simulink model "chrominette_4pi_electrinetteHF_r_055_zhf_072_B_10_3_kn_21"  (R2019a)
settings: Solver=VariableStepAuto  StartTime=0.0  StopTime=2329176.80  FixedStep=0.2  RelTol=1e-6

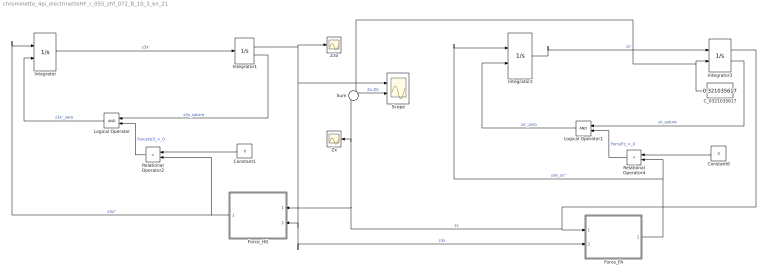
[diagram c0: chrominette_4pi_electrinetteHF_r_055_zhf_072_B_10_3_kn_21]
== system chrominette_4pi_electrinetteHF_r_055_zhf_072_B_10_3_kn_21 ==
  C_0321035617 : Constant  Value=0.321035617
  Constant1 : Constant  Value=0
  Constant6 : Constant  Value=0
  Force_FA : Subsystem
  Force_HG : Subsystem
  Integrator : Integrator  ExternalReset=level
  Integrator1 : Integrator  LimitOutput=on  UpperSaturationLimit=0  ShowSaturationPort=on  ZeroCross=off
  Integrator2 : Integrator  ExternalReset=level
  Integrator3 : Integrator  InitialConditionSource=external  LimitOutput=on  LowerSaturationLimit=0.321035617  ShowSaturationPort=on  ZeroCross=off
  Logical Operator : Logic  AllPortsSameDT=off  OutDataTypeStr=boolean
  Logical Operator1 : Logic  AllPortsSameDT=off  OutDataTypeStr=boolean
  Relational Operator2 : RelationalOperator  Operator=<  OutDataTypeStr=boolean  RndMeth=Simplest
  Relational Operator4 : RelationalOperator  Operator=>  OutDataTypeStr=boolean  RndMeth=Simplest
  Scope : Scope  NumInputPorts=2
  Sum : Sum  Inputs=-+
  Z3x : Scope
  Zx : Scope
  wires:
  Integrator/1 -> Integrator1/1  "z3x'"
  Integrator1/1 -> Scope/1, Force_FA/2(In2), Force_HG/2(In2), Z3x/1  "z3x"
  Force_HG/1(Out1) -> Relational Operator2/2, Integrator/1  "z3x''"
  Constant1/1 -> Relational Operator2/1
  Relational Operator2/1 -> Logical Operator/2  "ForceHz3_>_0"
  Constant6/1 -> Relational Operator4/1
  Integrator3/1 -> Force_HG/1(In1), Zx/1, Sum/2, Force_FA/1(In1)  "zx"
  Logical Operator1/1 -> Integrator2/2  "zx'_zero"
  Relational Operator4/1 -> Logical Operator1/2  "ForceFz_<_0"
  C_0321035617/1 -> Integrator3/2, Sum/1
  Force_FA/1(Out1) -> Integrator2/1, Relational Operator4/2  "pre_zx''"
  Integrator1/2 -> Logical Operator/1  "z3x_sature"
  Logical Operator/1 -> Integrator/2  "z3x'_zero"
  Integrator3/2 -> Logical Operator1/1  "zx_sature"
  Integrator2/1 -> Integrator3/1  "zx'"
  Sum/1 -> Scope/2  "Zx-Z0"

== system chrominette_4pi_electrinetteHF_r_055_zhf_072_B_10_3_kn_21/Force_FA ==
  In1 : Inport
  In2 : Inport  Port=2
  Add26 : Sum  Inputs=-+
  F_AG : Subsystem
  F_AH : Subsystem
  F_AI : Subsystem
  F_AJ : Subsystem
  F_FG : Subsystem
  F_FH : Subsystem
  F_FI : Subsystem
  F_FJ : Subsystem
  Scope14 : Scope
  Sum1 : Sum  Inputs=|+|-|+|-|-|+|-|+
  Z0_1 : Constant  Value=0.321035617
  Out1 : Outport
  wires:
  Sum1/1 -> Scope14/1, Out1/1  "pre_zx''"
  In1/1 -> F_AI/1(In1), F_AJ/1(In1), F_AG/1(In1), F_AH/1(In1), F_FH/1(In1), F_FG/1(In1), F_FJ/1(In1), F_FI/1(In1)
  F_FG/1(Out1) -> Sum1/5
  F_FI/1(Out1) -> Sum1/1
  Z0_1/1 -> Add26/2  "Z0"
  In2/1 -> Add26/1  "z3"
  Add26/1 -> F_FH/2(In2), F_AG/2(In2), F_FG/2(In2), F_AH/2(In2)  "z0 - z3"
  F_AI/1(Out1) -> Sum1/2
  F_FJ/1(Out1) -> Sum1/3
  F_AJ/1(Out1) -> Sum1/4
  F_AH/1(Out1) -> Sum1/8
  F_FH/1(Out1) -> Sum1/7
  F_AG/1(Out1) -> Sum1/6

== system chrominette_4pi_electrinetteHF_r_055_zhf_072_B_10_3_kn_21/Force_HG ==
  In1 : Inport
  In2 : Inport  Port=2
  F_HA : Subsystem
  F_HF : Subsystem
  F_HI : Subsystem
  F_HJ : Subsystem
  Scope : Scope
  Sum : Sum  Inputs=|+|-|+|-
  Out1 : Outport
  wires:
  In2/1 -> F_HJ/2(In2), F_HI/2(In2), F_HF/2(In2), F_HA/2(In2)
  In1/1 -> F_HJ/1(In1), F_HI/1(In1), F_HF/1(In1), F_HA/1(In1)
  Sum/1 -> Out1/1, Scope/1  "pre_z3x''"
  F_HA/1(Out1) -> Sum/1
  F_HF/1(Out1) -> Sum/2
  F_HI/1(Out1) -> Sum/3
  F_HJ/1(Out1) -> Sum/4

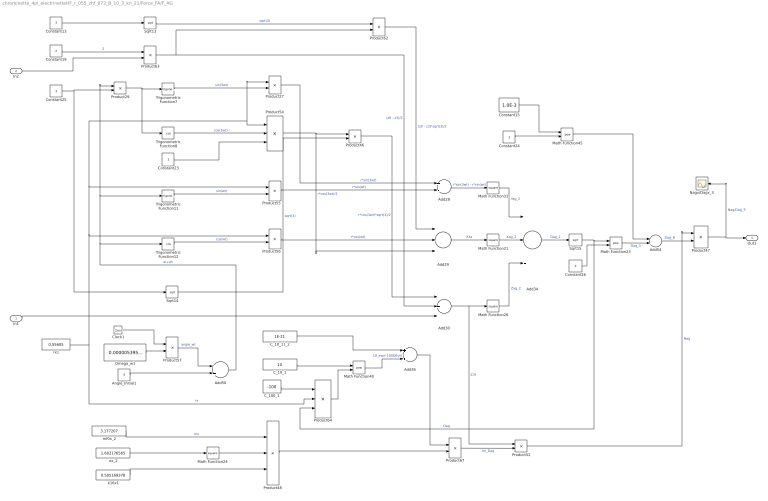
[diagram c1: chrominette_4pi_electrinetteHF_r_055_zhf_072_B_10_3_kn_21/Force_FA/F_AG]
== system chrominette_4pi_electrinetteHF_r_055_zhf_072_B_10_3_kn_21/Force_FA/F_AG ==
  In1 : Inport
  In2 : Inport  Port=2
  Add28 : Sum  Inputs=+-
  Add29 : Sum  Inputs=-++
  Add30 : Sum  Inputs=+++
  Add34 : Sum  Inputs=+++
  Add36 : Sum
  Add50 : Sum
  Add54 : Sum
  Angle_Initial1 : Constant  Value=0
  C_100_1 : Constant  Value=-100
  C_10_1 : Constant  Value=10
  C_10_11_2 : Constant  Value=1E-21
  Clock1 : Clock
  Constant{13,24..26} (4 alike) : Constant  Value=3
  Constant15 : Constant  Value=1.0E-3
  Constant19 : Constant  Value=2
  Constant23 : Constant  Value=2
  Math Function{21,24,26,31} (4 alike) : Math  Operator=square
  Math Function23 : Math  Operator=pow
  Math Function40 : Math  Operator=pow
  Math Function45 : Math  Operator=pow
  Nagx/Dagx_3 : Scope
  Omega_w1 : Constant  Value=0.000005395198
  Product{27,55..56,62,67} (5 alike) : Product  Inputs=**
  Product{29,46,52,57} (4 alike) : Product
  Product47 : Product  Inputs=*/
  Product48 : Product  Inputs=/**
  Product54 : Product  Inputs=**/
  Product63 : Product  Inputs=/*
  Product64 : Product  Inputs=*/*
  Sqrt13 : Sqrt
  Sqrt14 : Sqrt
  Sqrt15 : Sqrt
  Trigonometric Function11 : Trigonometry
  Trigonometric Function12 : Trigonometry  Operator=cos
  Trigonometric Function7 : Trigonometry
  Trigonometric Function8 : Trigonometry  Operator=cos
  ex_2 : Constant  Value=1.602176565
  k16x1 : Constant  Value=0.505169378
  mf0x_2 : Constant  Value=3.177207
  rx1 : Constant  Value=0.55605
  Out1 : Outport
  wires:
  Product52/1 -> Product47/1  "Nag"
  Product29/1 -> Trigonometric Function8/1, Trigonometric Function7/1
  C_10_11_2/1 -> Add36/1
  Constant13/1 -> Sqrt13/1
  Add54/1 -> Product47/2  "Dag_B"
  Constant15/1 -> Math Function45/1
  Add29/1 -> Math Function21/1  "X3a"
  Constant25/1 -> Sqrt14/1, Product29/2
  Add34/1 -> Sqrt15/1  "Dag_2"
  Constant24/1 -> Math Function45/2
  Trigonometric Function11/1 -> Product55/2  "sin(wt)"
  Product54/1 -> Add29/3, Product46/1  "r*cos(3wt)/2"
  Constant23/1 -> Product54/3
  Product48/1 -> Product67/2
  Trigonometric Function12/1 -> Product56/2  "cos(wt)"
  Math Function40/1 -> Add36/2  "10_exp(-100Dfh/r)"
  Product64/1 -> Math Function40/2
  Trigonometric Function7/1 -> Product27/2  "sin(3wt)"
  Product47/1 -> Out1/1, Nagx/Dagx_3/1  "Nag/Dag_3"
  ex_2/1 -> Math Function24/1
  Product62/1 -> Add29/1  "(z0 - z3)*sqrt(3)/2"
  Product55/1 -> Add28/2  "r*sin(wt)"
  Clock1/1 -> Product57/1
  Product27/1 -> Add28/1  "r*sin(3wt)"
  Constant26/1 -> Math Function23/2
  Sqrt14/1 -> Product46/2  "sqrt(3)"
  Sqrt13/1 -> Product62/1  "sqrt(3)"
  Product57/1 -> Add50/1  "angle_wt"
  Math Function45/1 -> Add54/1
  Math Function23/1 -> Add54/2  "Dag_3"
  Constant19/1 -> Product63/1  "2"
  C_100_1/1 -> Product64/1
  Trigonometric Function8/1 -> Product54/2  "cos(3wt)"
  Product67/1 -> Product52/2  "kn_Dag"
  Sqrt15/1 -> Math Function23/1, Product64/3  "Dag"
  Product56/1 -> Add29/2  "r*cos(wt)"
  Add28/1 -> Math Function31/1  "r*sin(3wt) - r*sin(wt)"
  Angle_Initial1/1 -> Add50/2
  C_10_1/1 -> Math Function40/1
  Product46/1 -> Add30/1  "r*cos(3wt)*sqrt(3)/2"
  Product63/1 -> Add30/2, Product62/2  "(z0 - z3)/2"
  Math Function24/1 -> Product48/2
  Add36/1 -> Product67/1
  Omega_w1/1 -> Product57/2
  k16x1/1 -> Product48/3
  Math Function26/1 -> Add34/3  "Zag_2"
  mf0x_2/1 -> Product48/1  "mx"
  Math Function21/1 -> Add34/2  "Xag_2"
  Math Function31/1 -> Add34/1  "Yag_2"
  Add50/1 -> Trigonometric Function12/1, Trigonometric Function11/1, Product29/1  "ai+wt"
  rx1/1 -> Product56/1, Product55/1, Product27/1, Product54/1, Product64/2  "rx"
  In2/1 -> Product63/2
  Add30/1 -> Math Function26/1, Product52/1  "Z3f"
  In1/1 -> Add30/3

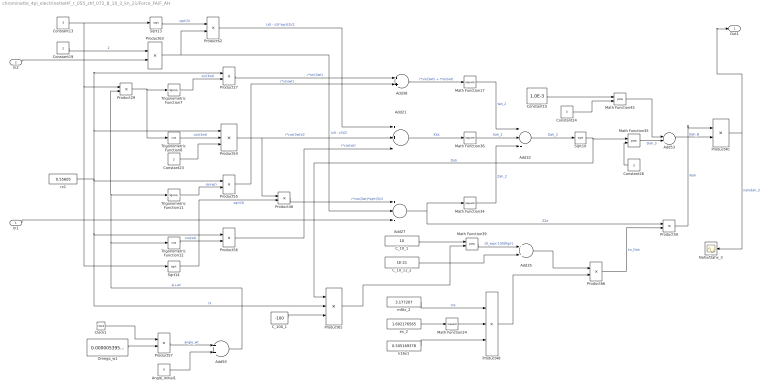
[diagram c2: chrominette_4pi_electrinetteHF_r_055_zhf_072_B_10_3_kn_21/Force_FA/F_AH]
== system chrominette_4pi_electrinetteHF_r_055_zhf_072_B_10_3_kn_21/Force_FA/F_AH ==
  In1 : Inport
  In2 : Inport  Port=2
  Add21 : Sum  Inputs=++-
  Add27 : Sum  Inputs=+--
  Add32 : Sum  Inputs=+++
  Add{35,38,50,53} (4 alike) : Sum
  Angle_Initial1 : Constant  Value=0
  C_100_1 : Constant  Value=-100
  C_10_1 : Constant  Value=10
  C_10_11_2 : Constant  Value=1E-21
  Clock1 : Clock
  Constant13 : Constant  Value=3
  Constant15 : Constant  Value=1.0E-3
  Constant19 : Constant  Value=2
  Constant23 : Constant  Value=2
  Constant24 : Constant  Value=3
  Constant26 : Constant  Value=3
  Math Function{17,24,34,36} (4 alike) : Math  Operator=square
  Math Function35 : Math  Operator=pow
  Math Function39 : Math  Operator=pow
  Math Function45 : Math  Operator=pow
  Nahx/Dahx_3 : Scope
  Omega_w1 : Constant  Value=0.000005395198
  Product{27,55..56,62,66} (5 alike) : Product  Inputs=**
  Product{29,46,50,57} (4 alike) : Product
  Product40 : Product  Inputs=*/
  Product48 : Product  Inputs=/**
  Product54 : Product  Inputs=**/
  Product63 : Product  Inputs=/*
  Product65 : Product  Inputs=*/*
  Sqrt10 : Sqrt
  Sqrt13 : Sqrt
  Sqrt14 : Sqrt
  Trigonometric Function11 : Trigonometry
  Trigonometric Function12 : Trigonometry  Operator=cos
  Trigonometric Function7 : Trigonometry
  Trigonometric Function8 : Trigonometry  Operator=cos
  ex_2 : Constant  Value=1.602176565
  k16x1 : Constant  Value=0.505169378
  mf0x_2 : Constant  Value=3.177207
  rx1 : Constant  Value=0.55605
  Out1 : Outport
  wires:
  Product50/1 -> Product40/1  "Nah"
  C_10_1/1 -> Math Function39/1
  Constant26/1 -> Math Function35/2
  Product27/1 -> Add38/1  "r*sin(3wt)"
  Product46/1 -> Add27/1  "r*cos(3wt)*sqrt(3)/2"
  Product65/1 -> Math Function39/2
  Math Function36/1 -> Add32/2  "Xah_2"
  Sqrt10/1 -> Product65/1, Math Function35/1  "Dah"
  Math Function24/1 -> Product48/2
  mf0x_2/1 -> Product48/1  "mx"
  Math Function17/1 -> Add32/1  "Yah_2"
  ex_2/1 -> Math Function24/1
  k16x1/1 -> Product48/3
  Add53/1 -> Product40/2  "Dah_B"
  Add27/1 -> Math Function34/1, Product50/1  "Z2a"
  Product54/1 -> Add21/2, Product46/1  "r*cos(3wt)/2"
  C_100_1/1 -> Product65/3
  Add38/1 -> Math Function17/1  "r*sin(3wt) + r*sin(wt)"
  Product55/1 -> Add38/2  "r*sin(wt)"
  Add32/1 -> Sqrt10/1  "Dah_2"
  Sqrt14/1 -> Product46/2  "sqrt(3)"
  Product62/1 -> Add21/1  "(z0 - z3)*sqrt(3)/2"
  Constant19/1 -> Product63/1  "2"
  Constant13/1 -> Product29/1, Sqrt14/1, Sqrt13/1
  Constant15/1 -> Math Function45/1
  Product63/1 -> Add27/2, Product62/2  "(z0 - z3)/2"
  Add35/1 -> Product66/1
  Sqrt13/1 -> Product62/1  "sqrt(3)"
  Math Function34/1 -> Add32/3  "Zah_2"
  Product29/1 -> Trigonometric Function8/1, Trigonometric Function7/1
  Add21/1 -> Math Function36/1  "X2a"
  Constant24/1 -> Math Function45/2
  Trigonometric Function11/1 -> Product55/2  "sin(wt)"
  Constant23/1 -> Product54/3
  Trigonometric Function8/1 -> Product54/2  "cos(3wt)"
  Trigonometric Function12/1 -> Product56/2  "cos(wt)"
  rx1/1 -> Product27/1, Product54/1, Product65/2, Product56/1, Product55/1  "rx"
  Trigonometric Function7/1 -> Product27/2  "sin(3wt)"
  Math Function39/1 -> Add35/1  "10_exp(-100Dfg/r)"
  Product56/1 -> Add21/3  "r*cos(wt)"
  Product48/1 -> Product66/2
  C_10_11_2/1 -> Add35/2
  Math Function35/1 -> Add53/2  "Dah_3"
  Product66/1 -> Product50/2  "kn_Dah"
  In2/1 -> Product63/2
  In1/1 -> Add27/3
  Math Function45/1 -> Add53/1
  Clock1/1 -> Product57/1
  Product57/1 -> Add50/1  "angle_wt"
  Omega_w1/1 -> Product57/2
  Angle_Initial1/1 -> Add50/2
  Add50/1 -> Trigonometric Function12/1, Product29/2, Trigonometric Function11/1  "ai+wt"
  Product40/1 -> Nahx/Dahx_3/1, Out1/1  "nah/dah_3"

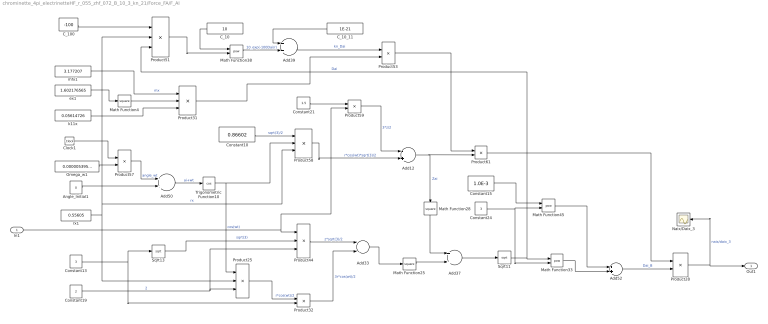
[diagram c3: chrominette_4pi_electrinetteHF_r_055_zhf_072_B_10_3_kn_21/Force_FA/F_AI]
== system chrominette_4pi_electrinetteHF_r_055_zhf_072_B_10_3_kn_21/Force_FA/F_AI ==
  In1 : Inport
  Add12 : Sum  Inputs=-+
  Add33 : Sum  Inputs=--
  Add{37,39,50,52} (4 alike) : Sum
  Angle_Initial1 : Constant  Value=0
  C_10 : Constant  Value=10
  C_100 : Constant  Value=-100
  C_10_11 : Constant  Value=1E-21
  Clock1 : Clock
  Constant10 : Constant  Value=0.86602
  Constant13 : Constant  Value=3
  Constant15 : Constant  Value=1.0E-3
  Constant19 : Constant  Value=2
  Constant21 : Constant  Value=1.5
  Constant24 : Constant  Value=3
  Math Function25 : Math  Operator=square
  Math Function28 : Math  Operator=square
  Math Function33 : Math  Operator=pow
  Math Function38 : Math  Operator=pow
  Math Function4 : Math  Operator=square
  Math Function45 : Math  Operator=pow
  Naix/Daix_3 : Scope
  Omega_w1 : Constant  Value=0.000005395198
  Product25 : Product  Inputs=**/
  Product28 : Product  Inputs=*/
  Product31 : Product  Inputs=/**
  Product{32,53,57,59,61} (5 alike) : Product
  Product44 : Product  Inputs=**/
  Product51 : Product  Inputs=*/*
  Product58 : Product  Inputs=3
  Sqrt11 : Sqrt
  Sqrt13 : Sqrt
  Trigonometric Function10 : Trigonometry  Operator=cos
  ex1 : Constant  Value=1.602176565
  k11x : Constant  Value=0.05614726
  mfx1 : Constant  Value=3.177207
  rx1 : Constant  Value=0.55605
  Out1 : Outport
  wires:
  Sqrt11/1 -> Product51/3, Math Function33/1  "Dai"
  Constant13/1 -> Sqrt13/1, Product32/2
  Constant15/1 -> Math Function45/1
  Product25/1 -> Product32/1  "r*cos(wt)/2"
  Add33/1 -> Math Function25/1
  k11x/1 -> Product31/3
  Product59/1 -> Add12/1  "3*z/2"
  Add12/1 -> Math Function28/1, Product61/2  "Zai"
  Product32/1 -> Add33/2  "3r*cos(wt)/2"
  Product61/1 -> Product28/1
  Constant24/1 -> Math Function33/2, Math Function45/2
  Add52/1 -> Product28/2  "Dai_B"
  C_10_11/1 -> Add39/1
  Add39/1 -> Product53/1  "kn_Dai"
  Math Function25/1 -> Add37/2
  Math Function28/1 -> Add37/1
  Math Function4/1 -> Product31/2
  Clock1/1 -> Product57/1
  Product58/1 -> Add12/2  "r*cos(wt)*sqrt(3)/2"
  Sqrt13/1 -> Product44/2  "sqrt(3)"
  C_100/1 -> Product51/1
  Product57/1 -> Add50/1  "angle_wt"
  Product44/1 -> Add33/1  "z*sqrt(3)/2"
  Math Function45/1 -> Add52/1
  Math Function33/1 -> Add52/2
  ex1/1 -> Math Function4/1
  Constant19/1 -> Product25/3, Product44/3  "2"
  Trigonometric Function10/1 -> Product58/2, Product25/1  "cos(wt)"
  Add50/1 -> Trigonometric Function10/1  "ai+wt"
  Constant10/1 -> Product58/1  "sqrt(3)/2"
  Angle_Initial1/1 -> Add50/2
  Product53/1 -> Product61/1
  Product28/1 -> Out1/1, Naix/Daix_3/1  "naix/daix_3"
  Omega_w1/1 -> Product57/2
  Add37/1 -> Sqrt11/1
  C_10/1 -> Math Function38/1
  Math Function38/1 -> Add39/2  "10_exp(-100Dai/r)"
  Product51/1 -> Math Function38/2
  rx1/1 -> Product51/2, Product58/3, Product25/2  "rx"
  mfx1/1 -> Product31/1  "mx"
  Product31/1 -> Product53/2
  In1/1 -> Product59/2, Product44/1
  Constant21/1 -> Product59/1

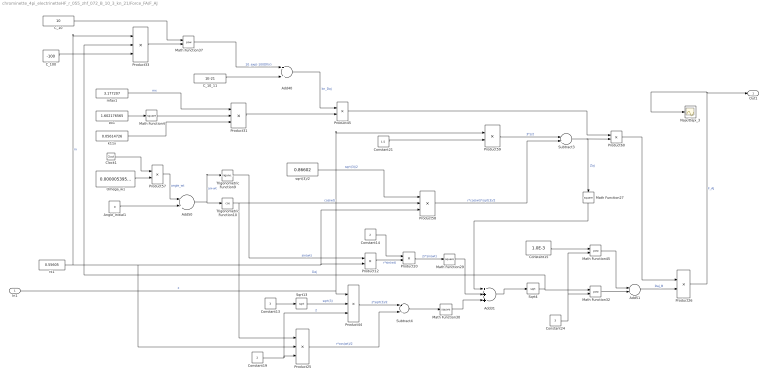
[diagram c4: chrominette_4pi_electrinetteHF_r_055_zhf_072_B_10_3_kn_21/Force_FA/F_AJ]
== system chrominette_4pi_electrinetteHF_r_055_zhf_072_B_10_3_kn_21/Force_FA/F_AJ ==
  In1 : Inport
  Add31 : Sum  Inputs=+++
  Add40 : Sum
  Add50 : Sum
  Add51 : Sum
  Angle_Initial1 : Constant  Value=0
  C_10 : Constant  Value=10
  C_100 : Constant  Value=-100
  C_10_11 : Constant  Value=1E-21
  Clock1 : Clock
  Constant13 : Constant  Value=3
  Constant14 : Constant  Value=2
  Constant15 : Constant  Value=1.0E-3
  Constant19 : Constant  Value=2
  Constant21 : Constant  Value=1.5
  Constant24 : Constant  Value=3
  Math Function{4,27,29..30} (4 alike) : Math  Operator=square
  Math Function32 : Math  Operator=pow
  Math Function37 : Math  Operator=pow
  Math Function45 : Math  Operator=pow
  Najx/Dajx_3 : Scope
  Omega_w1 : Constant  Value=0.000005395198
  Product{12,20,45,57,59..60} (6 alike) : Product
  Product25 : Product  Inputs=**/
  Product26 : Product  Inputs=*/
  Product31 : Product  Inputs=/**
  Product33 : Product  Inputs=/**
  Product44 : Product  Inputs=**/
  Product58 : Product  Inputs=3
  Sqrt13 : Sqrt
  Sqrt4 : Sqrt
  Subtract3 : Sum
  Subtract4 : Sum  Inputs=--
  Trigonometric Function10 : Trigonometry  Operator=cos
  Trigonometric Function9 : Trigonometry
  ex1 : Constant  Value=1.602176565
  k11x : Constant  Value=0.05614726
  mfax1 : Constant  Value=3.177207
  rx1 : Constant  Value=0.55605
  sqrt(3)/2 : Constant  Value=0.86602
  Out1 : Outport
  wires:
  Subtract4/1 -> Math Function30/1
  Math Function32/1 -> Add51/2
  Add40/1 -> Product45/1  "kn_Daj"
  Math Function45/1 -> Add51/1
  Product45/1 -> Product60/1
  Math Function4/1 -> Product31/2
  Math Function30/1 -> Add31/3
  Math Function37/1 -> Add40/1  "10_exp(-100Dfi/r)"
  Math Function29/1 -> Add31/2
  Clock1/1 -> Product57/1
  Product44/1 -> Subtract4/1  "z*sqrt(3)/2"
  sqrt(3)/2/1 -> Product58/1  "sqrt(3)/2"
  Add50/1 -> Trigonometric Function9/1, Trigonometric Function10/1  "ai+wt"
  Subtract3/1 -> Math Function27/1, Product60/2  "Zaj"
  C_100/1 -> Product33/3
  Trigonometric Function10/1 -> Product58/2, Product25/1  "cos(wt)"
  Product58/1 -> Subtract3/2  "r*cos(wt)*sqrt(3)/2"
  Add51/1 -> Product26/2  "Daj_B"
  Add31/1 -> Sqrt4/1
  C_10_11/1 -> Add40/2
  Product31/1 -> Product45/2
  Constant21/1 -> Product59/2
  Product57/1 -> Add50/1  "angle_wt"
  C_10/1 -> Math Function37/1
  mfax1/1 -> Product31/1  "mx"
  Constant19/1 -> Product25/3, Product44/3  "2"
  Constant13/1 -> Sqrt13/1
  Product33/1 -> Math Function37/2
  Constant15/1 -> Math Function45/1
  Product59/1 -> Subtract3/1  "3*z/2"
  Omega_w1/1 -> Product57/2
  Sqrt13/1 -> Product44/2  "sqrt(3)"
  k11x/1 -> Product31/3
  ex1/1 -> Math Function4/1
  Product12/1 -> Product20/2  "r*sin(wt)"
  Math Function27/1 -> Add31/1
  Constant24/1 -> Math Function32/2, Math Function45/2
  Constant14/1 -> Product20/1
  Trigonometric Function9/1 -> Product12/1  "sin(wt)"
  Product25/1 -> Subtract4/2  "r*cos(wt)/2"
  rx1/1 -> Product33/1, Product25/2, Product12/2, Product58/3  "rx"
  Product20/1 -> Math Function29/1  "2r*sin(wt)"
  Angle_Initial1/1 -> Add50/2
  Product26/1 -> Out1/1, Najx/Dajx_3/1  "F_AJ"
  Sqrt4/1 -> Product33/2, Math Function32/1  "Daj"
  In1/1 -> Product44/1, Product59/1  "z"
  Product60/1 -> Product26/1

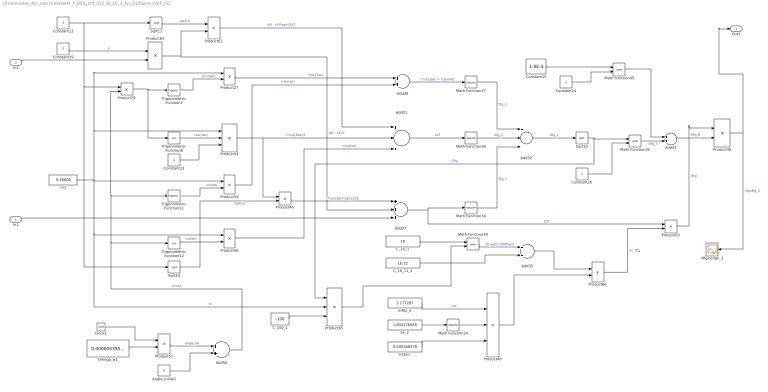
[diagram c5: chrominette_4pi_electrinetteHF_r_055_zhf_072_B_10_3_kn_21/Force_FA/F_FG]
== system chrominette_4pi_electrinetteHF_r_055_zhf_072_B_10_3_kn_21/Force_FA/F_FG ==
  In1 : Inport
  In2 : Inport  Port=2
  Add21 : Sum  Inputs=+-+
  Add27 : Sum  Inputs=+++
  Add32 : Sum  Inputs=+++
  Add{35,38,50,53} (4 alike) : Sum
  Angle_Initial1 : Constant  Value=0
  C_100_1 : Constant  Value=-100
  C_10_1 : Constant  Value=10
  C_10_11_2 : Constant  Value=1E-21
  Clock1 : Clock
  Constant13 : Constant  Value=3
  Constant15 : Constant  Value=1.0E-3
  Constant19 : Constant  Value=2
  Constant23 : Constant  Value=2
  Constant24 : Constant  Value=3
  Constant26 : Constant  Value=3
  Math Function{17,24,34,36} (4 alike) : Math  Operator=square
  Math Function35 : Math  Operator=pow
  Math Function39 : Math  Operator=pow
  Math Function45 : Math  Operator=pow
  Nfgx/Dfgx_3 : Scope
  Omega_w1 : Constant  Value=0.000005395198
  Product{27,55..56,62,66} (5 alike) : Product  Inputs=**
  Product{29,46,50,57} (4 alike) : Product
  Product40 : Product  Inputs=*/
  Product48 : Product  Inputs=/**
  Product54 : Product  Inputs=**/
  Product63 : Product  Inputs=/*
  Product65 : Product  Inputs=*/*
  Sqrt10 : Sqrt
  Sqrt13 : Sqrt
  Sqrt14 : Sqrt
  Trigonometric Function11 : Trigonometry
  Trigonometric Function12 : Trigonometry  Operator=cos
  Trigonometric Function7 : Trigonometry
  Trigonometric Function8 : Trigonometry  Operator=cos
  ex_2 : Constant  Value=1.602176565
  k16x1 : Constant  Value=0.505169378
  mf0x_2 : Constant  Value=3.177207
  rx1 : Constant  Value=0.55605
  Out1 : Outport
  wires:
  Product50/1 -> Product40/1  "Nfg"
  C_10_1/1 -> Math Function39/1
  Constant26/1 -> Math Function35/2
  Product27/1 -> Add38/1  "r*sin(3wt)"
  Product46/1 -> Add27/1  "r*cos(3wt)*sqrt(3)/2"
  Product65/1 -> Math Function39/2
  Math Function36/1 -> Add32/2  "Xfg_2"
  Sqrt10/1 -> Product65/1, Math Function35/1  "Dfg"
  Math Function24/1 -> Product48/2
  mf0x_2/1 -> Product48/1  "mx"
  Math Function17/1 -> Add32/1  "Yfg_2"
  ex_2/1 -> Math Function24/1
  k16x1/1 -> Product48/3
  Add53/1 -> Product40/2  "Dfg_B"
  Add27/1 -> Math Function34/1, Product50/1  "Z2f"
  Product54/1 -> Add21/2, Product46/1  "r*cos(3wt)/2"
  C_100_1/1 -> Product65/3
  Add38/1 -> Math Function17/1  "r*sin(3wt) + r*sin(wt)"
  Product55/1 -> Add38/2  "r*sin(wt)"
  Add32/1 -> Sqrt10/1  "Dfg_2"
  Sqrt14/1 -> Product46/2  "sqrt(3)"
  Product62/1 -> Add21/1  "(z0 - z3)*sqrt(3)/2"
  Constant19/1 -> Product63/1  "2"
  Constant13/1 -> Product29/1, Sqrt14/1, Sqrt13/1
  Constant15/1 -> Math Function45/1
  Product63/1 -> Add27/2, Product62/2  "(z0 - z3)/2"
  Add35/1 -> Product66/1
  Sqrt13/1 -> Product62/1  "sqrt(3)"
  Math Function34/1 -> Add32/3  "Zfg_2"
  Product29/1 -> Trigonometric Function8/1, Trigonometric Function7/1
  Add21/1 -> Math Function36/1  "X2f"
  Constant24/1 -> Math Function45/2
  Trigonometric Function11/1 -> Product55/2  "sin(wt)"
  Constant23/1 -> Product54/3
  Trigonometric Function8/1 -> Product54/2  "cos(3wt)"
  Trigonometric Function12/1 -> Product56/2  "cos(wt)"
  rx1/1 -> Product27/1, Product54/1, Product65/2, Product56/1, Product55/1  "rx"
  Trigonometric Function7/1 -> Product27/2  "sin(3wt)"
  Math Function39/1 -> Add35/1  "10_exp(-100Dfg/r)"
  Product56/1 -> Add21/3  "r*cos(wt)"
  Product48/1 -> Product66/2
  C_10_11_2/1 -> Add35/2
  Math Function35/1 -> Add53/2  "Dfg_3"
  Product66/1 -> Product50/2  "kn_Dfg"
  In2/1 -> Product63/2
  In1/1 -> Add27/3
  Math Function45/1 -> Add53/1
  Clock1/1 -> Product57/1
  Product57/1 -> Add50/1  "angle_wt"
  Omega_w1/1 -> Product57/2
  Angle_Initial1/1 -> Add50/2
  Add50/1 -> Trigonometric Function12/1, Product29/2, Trigonometric Function11/1  "ai+wt"
  Product40/1 -> Nfgx/Dfgx_3/1, Out1/1  "nfg/dfg_3"

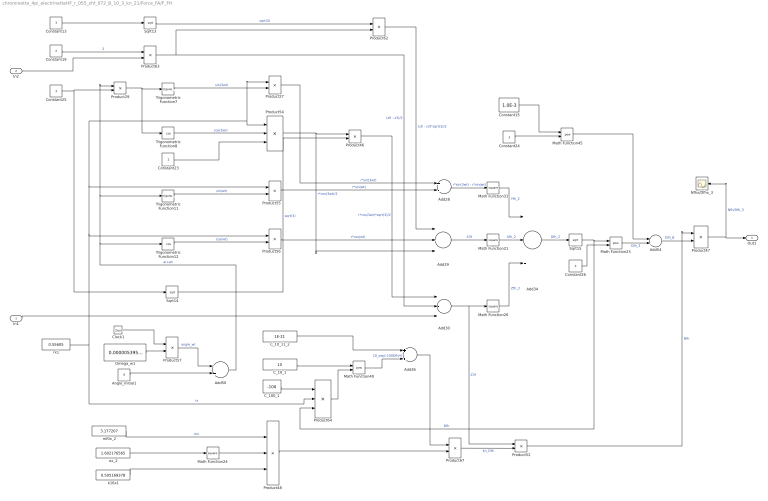
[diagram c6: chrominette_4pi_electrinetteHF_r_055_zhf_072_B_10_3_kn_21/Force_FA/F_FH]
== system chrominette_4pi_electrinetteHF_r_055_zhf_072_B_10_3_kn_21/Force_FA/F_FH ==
  In1 : Inport
  In2 : Inport  Port=2
  Add28 : Sum  Inputs=+-
  Add29 : Sum  Inputs=+++
  Add30 : Sum  Inputs=+--
  Add34 : Sum  Inputs=+++
  Add36 : Sum
  Add50 : Sum
  Add54 : Sum
  Angle_Initial1 : Constant  Value=0
  C_100_1 : Constant  Value=-100
  C_10_1 : Constant  Value=10
  C_10_11_2 : Constant  Value=1E-21
  Clock1 : Clock
  Constant{13,24..26} (4 alike) : Constant  Value=3
  Constant15 : Constant  Value=1.0E-3
  Constant19 : Constant  Value=2
  Constant23 : Constant  Value=2
  Math Function{21,24,26,31} (4 alike) : Math  Operator=square
  Math Function23 : Math  Operator=pow
  Math Function40 : Math  Operator=pow
  Math Function45 : Math  Operator=pow
  Nfhx/Dfhx_3 : Scope
  Omega_w1 : Constant  Value=0.000005395198
  Product{27,55..56,62,67} (5 alike) : Product  Inputs=**
  Product{29,46,52,57} (4 alike) : Product
  Product47 : Product  Inputs=*/
  Product48 : Product  Inputs=/**
  Product54 : Product  Inputs=**/
  Product63 : Product  Inputs=/*
  Product64 : Product  Inputs=*/*
  Sqrt13 : Sqrt
  Sqrt14 : Sqrt
  Sqrt15 : Sqrt
  Trigonometric Function11 : Trigonometry
  Trigonometric Function12 : Trigonometry  Operator=cos
  Trigonometric Function7 : Trigonometry
  Trigonometric Function8 : Trigonometry  Operator=cos
  ex_2 : Constant  Value=1.602176565
  k16x1 : Constant  Value=0.505169378
  mf0x_2 : Constant  Value=3.177207
  rx1 : Constant  Value=0.55605
  Out1 : Outport
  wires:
  Product52/1 -> Product47/1  "Nfh"
  Product29/1 -> Trigonometric Function8/1, Trigonometric Function7/1
  C_10_11_2/1 -> Add36/1
  Constant13/1 -> Sqrt13/1
  Add54/1 -> Product47/2  "Dfh_B"
  Constant15/1 -> Math Function45/1
  Add29/1 -> Math Function21/1  "X3f"
  Constant25/1 -> Sqrt14/1, Product29/2
  Add34/1 -> Sqrt15/1  "Dfh_2"
  Constant24/1 -> Math Function45/2
  Trigonometric Function11/1 -> Product55/2  "sin(wt)"
  Product54/1 -> Add29/3, Product46/1  "r*cos(3wt)/2"
  Constant23/1 -> Product54/3
  Product48/1 -> Product67/2
  Trigonometric Function12/1 -> Product56/2  "cos(wt)"
  Math Function40/1 -> Add36/2  "10_exp(-100Dfh/r)"
  Product64/1 -> Math Function40/2
  Trigonometric Function7/1 -> Product27/2  "sin(3wt)"
  Product47/1 -> Out1/1, Nfhx/Dfhx_3/1  "Nfh/Dfh_3"
  ex_2/1 -> Math Function24/1
  Product62/1 -> Add29/1  "(z0 - z3)*sqrt(3)/2"
  Product55/1 -> Add28/2  "r*sin(wt)"
  Clock1/1 -> Product57/1
  Product27/1 -> Add28/1  "r*sin(3wt)"
  Constant26/1 -> Math Function23/2
  Sqrt14/1 -> Product46/2  "sqrt(3)"
  Sqrt13/1 -> Product62/1  "sqrt(3)"
  Product57/1 -> Add50/1  "angle_wt"
  Math Function45/1 -> Add54/1
  Math Function23/1 -> Add54/2  "Dfh_3"
  Constant19/1 -> Product63/1  "2"
  C_100_1/1 -> Product64/1
  Trigonometric Function8/1 -> Product54/2  "cos(3wt)"
  Product67/1 -> Product52/2  "kn_Dfh"
  Sqrt15/1 -> Math Function23/1, Product64/3  "Dfh"
  Product56/1 -> Add29/2  "r*cos(wt)"
  Add28/1 -> Math Function31/1  "r*sin(3wt) - r*sin(wt)"
  Angle_Initial1/1 -> Add50/2
  C_10_1/1 -> Math Function40/1
  Product46/1 -> Add30/1  "r*cos(3wt)*sqrt(3)/2"
  Product63/1 -> Add30/2, Product62/2  "(z0 - z3)/2"
  Math Function24/1 -> Product48/2
  Add36/1 -> Product67/1
  Omega_w1/1 -> Product57/2
  k16x1/1 -> Product48/3
  Math Function26/1 -> Add34/3  "Zfh_2"
  mf0x_2/1 -> Product48/1  "mx"
  Math Function21/1 -> Add34/2  "Xfh_2"
  Math Function31/1 -> Add34/1  "Yfh_2"
  Add50/1 -> Trigonometric Function12/1, Trigonometric Function11/1, Product29/1  "ai+wt"
  rx1/1 -> Product56/1, Product55/1, Product27/1, Product54/1, Product64/2  "rx"
  In2/1 -> Product63/2
  Add30/1 -> Math Function26/1, Product52/1  "Z3f"
  In1/1 -> Add30/3

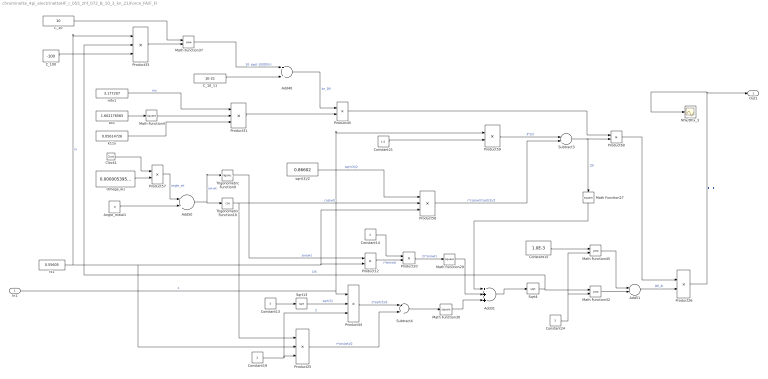
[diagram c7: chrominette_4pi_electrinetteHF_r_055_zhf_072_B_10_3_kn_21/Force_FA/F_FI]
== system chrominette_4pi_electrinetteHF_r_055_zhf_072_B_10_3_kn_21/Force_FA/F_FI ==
  In1 : Inport
  Add31 : Sum  Inputs=+++
  Add40 : Sum
  Add50 : Sum
  Add51 : Sum
  Angle_Initial1 : Constant  Value=0
  C_10 : Constant  Value=10
  C_100 : Constant  Value=-100
  C_10_11 : Constant  Value=1E-21
  Clock1 : Clock
  Constant13 : Constant  Value=3
  Constant14 : Constant  Value=2
  Constant15 : Constant  Value=1.0E-3
  Constant19 : Constant  Value=2
  Constant21 : Constant  Value=1.5
  Constant24 : Constant  Value=3
  Math Function{4,27,29..30} (4 alike) : Math  Operator=square
  Math Function32 : Math  Operator=pow
  Math Function37 : Math  Operator=pow
  Math Function45 : Math  Operator=pow
  Nfix/Dfix_3 : Scope
  Omega_w1 : Constant  Value=0.000005395198
  Product{12,20,45,57,59..60} (6 alike) : Product
  Product25 : Product  Inputs=**/
  Product26 : Product  Inputs=*/
  Product31 : Product  Inputs=/**
  Product33 : Product  Inputs=/**
  Product44 : Product  Inputs=**/
  Product58 : Product  Inputs=3
  Sqrt13 : Sqrt
  Sqrt4 : Sqrt
  Subtract3 : Sum  Inputs=-+
  Subtract4 : Sum  Inputs=-+
  Trigonometric Function10 : Trigonometry  Operator=cos
  Trigonometric Function9 : Trigonometry
  ex1 : Constant  Value=1.602176565
  k11x : Constant  Value=0.05614726
  mfx1 : Constant  Value=3.177207
  rx1 : Constant  Value=0.55605
  sqrt(3)/2 : Constant  Value=0.86602
  Out1 : Outport
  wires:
  Subtract4/1 -> Math Function30/1
  Math Function32/1 -> Add51/2
  Add40/1 -> Product45/1  "kn_Dfi"
  Math Function45/1 -> Add51/1
  Product45/1 -> Product60/1
  Math Function4/1 -> Product31/2
  Math Function30/1 -> Add31/3
  Math Function37/1 -> Add40/1  "10_exp(-100Dfi/r)"
  Math Function29/1 -> Add31/2
  Clock1/1 -> Product57/1
  Product44/1 -> Subtract4/1  "z*sqrt(3)/2"
  sqrt(3)/2/1 -> Product58/1  "sqrt(3)/2"
  Add50/1 -> Trigonometric Function9/1, Trigonometric Function10/1  "ai+wt"
  Subtract3/1 -> Math Function27/1, Product60/2  "Zfi"
  C_100/1 -> Product33/3
  Trigonometric Function10/1 -> Product58/2, Product25/1  "cos(wt)"
  Product58/1 -> Subtract3/2  "r*cos(wt)*sqrt(3)/2"
  Add51/1 -> Product26/2  "Dfi_B"
  Add31/1 -> Sqrt4/1
  C_10_11/1 -> Add40/2
  Product31/1 -> Product45/2
  Constant21/1 -> Product59/2
  Product57/1 -> Add50/1  "angle_wt"
  C_10/1 -> Math Function37/1
  mfx1/1 -> Product31/1  "mx"
  Constant19/1 -> Product25/3, Product44/3  "2"
  Constant13/1 -> Sqrt13/1
  Product33/1 -> Math Function37/2
  Constant15/1 -> Math Function45/1
  Product59/1 -> Subtract3/1  "3*z/2"
  Omega_w1/1 -> Product57/2
  Sqrt13/1 -> Product44/2  "sqrt(3)"
  k11x/1 -> Product31/3
  ex1/1 -> Math Function4/1
  Product12/1 -> Product20/2  "r*sin(wt)"
  Math Function27/1 -> Add31/1
  Constant24/1 -> Math Function32/2, Math Function45/2
  Constant14/1 -> Product20/1
  Trigonometric Function9/1 -> Product12/1  "sin(wt)"
  Product25/1 -> Subtract4/2  "r*cos(wt)/2"
  rx1/1 -> Product33/1, Product25/2, Product12/2, Product58/3  "rx"
  Product20/1 -> Math Function29/1  "2r*sin(wt)"
  Angle_Initial1/1 -> Add50/2
  Product26/1 -> Out1/1, Nfix/Dfix_3/1  "F_FI"
  Sqrt4/1 -> Product33/2, Math Function32/1  "Dfi"
  In1/1 -> Product44/1, Product59/1  "z"
  Product60/1 -> Product26/1

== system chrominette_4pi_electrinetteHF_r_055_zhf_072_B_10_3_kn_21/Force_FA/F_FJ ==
  In1 : Inport
  Add{12,37,39,50,52} (5 alike) : Sum
  Add33 : Sum  Inputs=-+
  Angle_Initial1 : Constant  Value=0
  C_10 : Constant  Value=10
  C_100 : Constant  Value=-100
  C_10_11 : Constant  Value=1E-21
  Clock1 : Clock
  Constant10 : Constant  Value=0.86602
  Constant13 : Constant  Value=3
  Constant15 : Constant  Value=1.0E-3
  Constant19 : Constant  Value=2
  Constant21 : Constant  Value=1.5
  Constant24 : Constant  Value=3
  Math Function25 : Math  Operator=square
  Math Function28 : Math  Operator=square
  Math Function33 : Math  Operator=pow
  Math Function38 : Math  Operator=pow
  Math Function4 : Math  Operator=square
  Math Function45 : Math  Operator=pow
  Nfjx/Dfjx_3 : Scope
  Omega_w1 : Constant  Value=0.000005395198
  Product25 : Product  Inputs=**/
  Product28 : Product  Inputs=*/
  Product31 : Product  Inputs=/**
  Product{32,53,57,59,61} (5 alike) : Product
  Product44 : Product  Inputs=**/
  Product51 : Product  Inputs=*/*
  Product58 : Product  Inputs=3
  Sqrt11 : Sqrt
  Sqrt13 : Sqrt
  Trigonometric Function10 : Trigonometry  Operator=cos
  ex1 : Constant  Value=1.602176565
  k11x : Constant  Value=0.05614726
  mfx1 : Constant  Value=3.177207
  rx1 : Constant  Value=0.55605
  Out1 : Outport
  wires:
  Sqrt11/1 -> Product51/3, Math Function33/1  "Dfj"
  Constant13/1 -> Sqrt13/1, Product32/2
  Constant15/1 -> Math Function45/1
  Product25/1 -> Product32/1  "r*cos(wt)/2"
  Add33/1 -> Math Function25/1
  k11x/1 -> Product31/3
  Product59/1 -> Add12/1  "3*z/2"
  Add12/1 -> Math Function28/1, Product61/2  "Zfj"
  Product32/1 -> Add33/2  "3r*cos(wt)/2"
  Product61/1 -> Product28/1
  Constant24/1 -> Math Function33/2, Math Function45/2
  Add52/1 -> Product28/2  "Dfj_B"
  C_10_11/1 -> Add39/1
  Add39/1 -> Product53/1  "kn_Dfj"
  Math Function25/1 -> Add37/2
  Math Function28/1 -> Add37/1
  Math Function4/1 -> Product31/2
  Clock1/1 -> Product57/1
  Product58/1 -> Add12/2  "r*cos(wt)*sqrt(3)/2"
  Sqrt13/1 -> Product44/2  "sqrt(3)"
  C_100/1 -> Product51/1
  Product57/1 -> Add50/1  "angle_wt"
  Product44/1 -> Add33/1  "z*sqrt(3)/2"
  Math Function45/1 -> Add52/1
  Math Function33/1 -> Add52/2
  ex1/1 -> Math Function4/1
  Constant19/1 -> Product25/3, Product44/3  "2"
  Trigonometric Function10/1 -> Product58/2, Product25/1  "cos(wt)"
  Add50/1 -> Trigonometric Function10/1  "ai+wt"
  Constant10/1 -> Product58/1  "sqrt(3)/2"
  Angle_Initial1/1 -> Add50/2
  Product53/1 -> Product61/1
  Product28/1 -> Out1/1, Nfjx/Dfjx_3/1  "nfjx/dfjx_3"
  Omega_w1/1 -> Product57/2
  Add37/1 -> Sqrt11/1
  C_10/1 -> Math Function38/1
  Math Function38/1 -> Add39/2  "10_exp(-100Dfj/r)"
  Product51/1 -> Math Function38/2
  rx1/1 -> Product51/2, Product58/3, Product25/2  "rx"
  mfx1/1 -> Product31/1  "mx"
  Product31/1 -> Product53/2
  In1/1 -> Product59/2, Product44/1
  Constant21/1 -> Product59/1

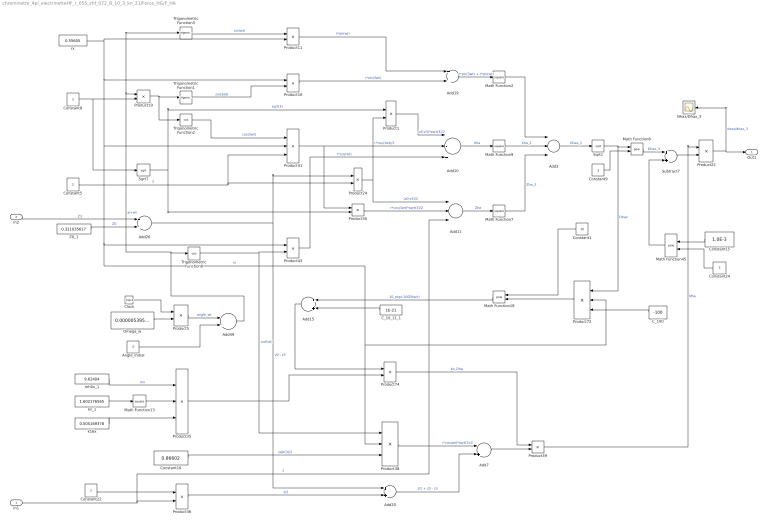
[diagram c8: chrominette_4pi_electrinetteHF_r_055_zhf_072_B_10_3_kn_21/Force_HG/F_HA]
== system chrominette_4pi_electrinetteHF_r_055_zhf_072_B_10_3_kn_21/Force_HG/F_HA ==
  In1 : Inport
  In2 : Inport  Port=2
  Add10 : Sum  Inputs=--+
  Add11 : Sum  Inputs=+-+
  Add{15,19..20,49} (4 alike) : Sum
  Add26 : Sum  Inputs=-+
  Add3 : Sum  Inputs=+++
  Add7 : Sum  Inputs=-+
  Angle_Initial : Constant  Value=0
  C_100 : Constant  Value=-100
  C_10_11_1 : Constant  Value=1E-21
  Clock : Clock
  Constant1 : Constant  Value=10
  Constant15 : Constant  Value=1.0E-3
  Constant16 : Constant  Value=0.86602
  Constant22 : Constant  Value=2
  Constant24 : Constant  Value=3
  Constant5 : Constant  Value=2
  Constant8 : Constant  Value=3
  Constant9 : Constant  Value=3
  Math Function{2,7,9,13} (4 alike) : Math  Operator=square
  Math Function18 : Math  Operator=pow
  Math Function45 : Math  Operator=pow
  Math Function8 : Math  Operator=pow
  Nhax/Dhax_3 : Scope
  Omega_w : Constant  Value=0.000005395168
  Product{1,16,43,74} (4 alike) : Product  Inputs=**
  Product{5,11,19,30,39} (5 alike) : Product
  Product22 : Product  Inputs=*/
  Product24 : Product  Inputs=*/
  Product35 : Product  Inputs=/**
  Product36 : Product  Inputs=/*
  Product38 : Product  Inputs=***
  Product41 : Product  Inputs=**/
  Product72 : Product  Inputs=*/*
  Sqrt1 : Sqrt
  Sqrt7 : Sqrt
  Subtract7 : Sum
  Trigonometric Function1 : Trigonometry
  Trigonometric Function2 : Trigonometry  Operator=cos
  Trigonometric Function3 : Trigonometry
  Trigonometric Function6 : Trigonometry  Operator=cos
  Z0_1 : Constant  Value=0.321035617
  ex_1 : Constant  Value=1.602176565
  k16x : Constant  Value=0.505169378
  mh0x_1 : Constant  Value=9.62404
  rx : Constant  Value=0.55605
  Out1 : Outport
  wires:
  Product16/1 -> Add19/2  "r*sin(3wt)"
  Omega_w/1 -> Product5/2
  Subtract7/1 -> Product22/2
  Add20/1 -> Add7/2  "z/2 + z0 - z3"
  Math Function8/1 -> Subtract7/1  "Dhax_3"
  Product22/1 -> Nhax/Dhax_3/1, Out1/1  "nhax/dhax_3"
  k16x/1 -> Product35/3
  Product1/1 -> Add10/1  "(z0-z3)*sqrt(3)/2"
  Trigonometric Function6/1 -> Product38/1, Product43/2  "cos(wt)"
  Add11/1 -> Math Function7/1  "Zha"
  Product43/1 -> Add10/3  "r*cos(wt)"
  Product41/1 -> Add10/2, Product30/1  "r*cos(3wt)/2"
  Product11/1 -> Add19/1  "r*sin(wt)"
  Math Function13/1 -> Product35/2
  Math Function18/1 -> Add15/1  "10_exp(-100Dha/r)"
  Trigonometric Function2/1 -> Product41/1  "cos(3wt)"
  Math Function9/1 -> Add3/2  "Xha_2"
  Product36/1 -> Add20/2  "z/2"
  Product24/1 -> Add11/1, Product1/2  "(z0-z3)/2"
  Constant8/1 -> Sqrt7/1, Product19/2
  Product39/1 -> Product22/1  "Nha"
  ex_1/1 -> Math Function13/1
  Product74/1 -> Product39/1  "kn_Dha"
  Trigonometric Function1/1 -> Product16/2  "sin(3wt)"
  Add3/1 -> Sqrt1/1  "Dhax_2"
  Math Function7/1 -> Add3/3  "Zha_2"
  Constant22/1 -> Product36/1
  Product38/1 -> Add7/1  "r*cos(wt)*sqrt(3)/2"
  Math Function2/1 -> Add3/1
  rx/1 -> Product41/2, Product43/1, Product72/2, Product38/2, Product16/1, Product11/2  "rx"
  Clock/1 -> Product5/1
  Add10/1 -> Math Function9/1  "Xha"
  Product72/1 -> Math Function18/2
  Constant16/1 -> Product38/3  "sqrt(3)/2"
  Trigonometric Function3/1 -> Product11/1  "sin(wt)"
  Product19/1 -> Trigonometric Function2/1, Trigonometric Function1/1
  Constant5/1 -> Product41/3, Product24/2  "2"
  Add26/1 -> Product24/1, Add20/1  "z0 - z3"
  Angle_Initial/1 -> Add49/2
  Product35/1 -> Product74/2
  C_10_11_1/1 -> Add15/2
  mh0x_1/1 -> Product35/1  "mx"
  Add15/1 -> Product74/1
  Product5/1 -> Add49/1  "angle_wt"
  Sqrt1/1 -> Math Function8/1, Product72/1  "Dhax"
  Sqrt7/1 -> Product30/2, Product1/1  "sqrt(3)"
  Constant9/1 -> Math Function8/2
  Add19/1 -> Math Function2/1  "r*sin(3wt) + r*sin(wt)"
  Product30/1 -> Add11/2  "r*cos(3wt)*sqrt(3)/2"
  Add49/1 -> Trigonometric Function6/1, Trigonometric Function3/1, Product19/1  "ai+wt"
  Z0_1/1 -> Add26/2  "Z0"
  In2/1 -> Add26/1  "Z3"
  In1/1 -> Add11/3, Product36/2  "z"
  Add7/1 -> Product39/2
  C_100/1 -> Product72/3
  Constant1/1 -> Math Function18/1
  Constant15/1 -> Math Function45/1
  Constant24/1 -> Math Function45/2
  Math Function45/1 -> Subtract7/2

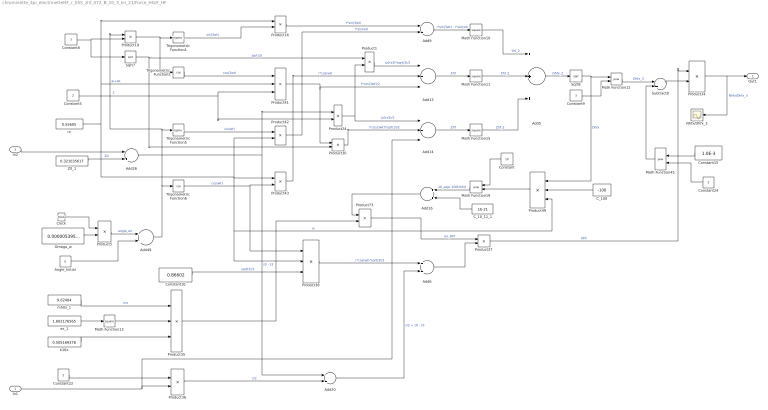
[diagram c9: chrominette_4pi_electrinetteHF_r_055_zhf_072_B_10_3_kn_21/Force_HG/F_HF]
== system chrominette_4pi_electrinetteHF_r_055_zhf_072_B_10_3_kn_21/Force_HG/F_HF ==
  In1 : Inport
  In2 : Inport  Port=2
  Add13 : Sum  Inputs=+++
  Add14 : Sum  Inputs=+-+
  Add{6,16,20,49} (4 alike) : Sum
  Add26 : Sum  Inputs=-+
  Add5 : Sum  Inputs=+++
  Add9 : Sum  Inputs=+-
  Angle_Initial : Constant  Value=0
  C_100 : Constant  Value=-100
  C_10_11_1 : Constant  Value=1E-21
  Clock : Clock
  Constant : Constant  Value=10
  Constant15 : Constant  Value=1.0E-3
  Constant16 : Constant  Value=0.86602
  Constant22 : Constant  Value=2
  Constant24 : Constant  Value=3
  Constant5 : Constant  Value=2
  Constant8 : Constant  Value=3
  Constant9 : Constant  Value=3
  Math Function{10..11,13,15} (4 alike) : Math  Operator=square
  Math Function12 : Math  Operator=pow
  Math Function19 : Math  Operator=pow
  Math Function45 : Math  Operator=pow
  Nhfx/Dhfx_3 : Scope
  Omega_w : Constant  Value=0.000005395168
  Product{1,16,42..43,73} (5 alike) : Product  Inputs=**
  Product{5,19,30,37} (4 alike) : Product
  Product24 : Product  Inputs=*/
  Product34 : Product  Inputs=*/
  Product35 : Product  Inputs=/**
  Product36 : Product  Inputs=/*
  Product38 : Product  Inputs=***
  Product41 : Product  Inputs=**/
  Product49 : Product  Inputs=**/
  Sqrt7 : Sqrt
  Sqrt8 : Sqrt
  Subtract8 : Sum
  Trigonometric Function1 : Trigonometry
  Trigonometric Function2 : Trigonometry  Operator=cos
  Trigonometric Function5 : Trigonometry
  Trigonometric Function6 : Trigonometry  Operator=cos
  Z0_1 : Constant  Value=0.321035617
  ex_1 : Constant  Value=1.602176565
  k16x : Constant  Value=0.505169378
  mh0x_1 : Constant  Value=9.62404
  rx : Constant  Value=0.55605
  Out1 : Outport
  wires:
  Constant15/1 -> Math Function45/1
  Product16/1 -> Add9/1  "r*sin(3wt)"
  Omega_w/1 -> Product5/2
  Add20/1 -> Add6/2  "z/2 + z0 - z3"
  k16x/1 -> Product35/3
  Sqrt8/1 -> Product49/1, Math Function12/1  "Dhfx"
  Product1/1 -> Add13/1  "(z0-z3)*sqrt(3)/2"
  Add9/1 -> Math Function10/1  "r*sin(3wt) - r*sin(wt)"
  Trigonometric Function6/1 -> Product38/1, Product43/2  "cos(wt)"
  Add5/1 -> Sqrt8/1  "Dhfx_2"
  Z0_1/1 -> Add26/2  "Z0"
  Product43/1 -> Add13/2  "r*cos(wt)"
  Product41/1 -> Product30/1, Add13/3  "r*cos(3wt)/2"
  Math Function13/1 -> Product35/2
  Trigonometric Function2/1 -> Product41/1  "cos(3wt)"
  Product36/1 -> Add20/2  "z/2"
  Product24/1 -> Add14/1, Product1/2  "(z0-z3)/2"
  Constant8/1 -> Sqrt7/1, Product19/2
  Product34/1 -> Out1/1, Nhfx/Dhfx_3/1  "Nhfx/Dhfx_3"
  ex_1/1 -> Math Function13/1
  Add49/1 -> Trigonometric Function6/1, Product19/1, Trigonometric Function5/1  "ai+wt"
  Product42/1 -> Add9/2  "r*sin(wt)"
  Trigonometric Function1/1 -> Product16/2  "sin(3wt)"
  Product73/1 -> Product37/1  "kn_Dhf"
  Trigonometric Function5/1 -> Product42/1  "sin(wt)"
  Math Function11/1 -> Add5/2  "Xhf_2"
  Add13/1 -> Math Function11/1  "Xhf"
  Constant22/1 -> Product36/1
  Product38/1 -> Add6/1  "r*cos(wt)*sqrt(3)/2"
  Constant24/1 -> Math Function45/2
  rx/1 -> Product38/2, Product49/3, Product42/2, Product43/1, Product16/1, Product41/2  "rx"
  Add16/1 -> Product73/1
  Clock/1 -> Product5/1
  Product37/1 -> Product34/1  "Nhf"
  Constant16/1 -> Product38/3  "sqrt(3)/2"
  Product19/1 -> Trigonometric Function2/1, Trigonometric Function1/1
  Constant5/1 -> Product24/2, Product41/3  "2"
  Add26/1 -> Add20/1, Product24/1  "z0 - z3"
  Angle_Initial/1 -> Add49/2
  Product35/1 -> Product73/2
  C_10_11_1/1 -> Add16/2
  mh0x_1/1 -> Product35/1  "mx"
  Add6/1 -> Product37/2
  Add14/1 -> Math Function15/1  "Zhf"
  Product49/1 -> Math Function19/2
  Product5/1 -> Add49/1  "angle_wt"
  Math Function19/1 -> Add16/1  "10_exp(-100Dhf/r)"
  Sqrt7/1 -> Product30/2, Product1/1  "sqrt(3)"
  Math Function15/1 -> Add5/3  "Zhf_2"
  Constant9/1 -> Math Function12/2
  Product30/1 -> Add14/2  "r*cos(3wt)*sqrt(3)/2"
  Math Function10/1 -> Add5/1  "Yhf_2"
  Math Function45/1 -> Subtract8/2
  Math Function12/1 -> Subtract8/1  "Dhfx_3"
  Subtract8/1 -> Product34/2
  In2/1 -> Add26/1
  In1/1 -> Add14/3, Product36/2
  C_100/1 -> Product49/2
  Constant/1 -> Math Function19/1

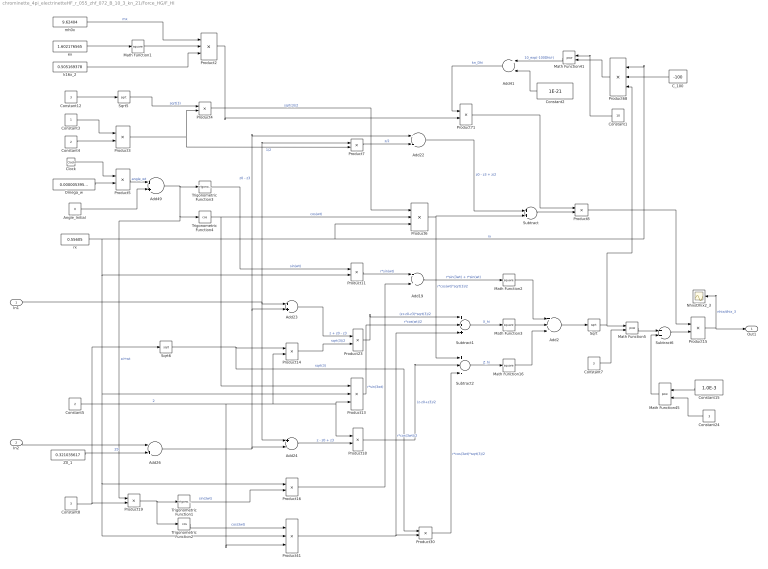
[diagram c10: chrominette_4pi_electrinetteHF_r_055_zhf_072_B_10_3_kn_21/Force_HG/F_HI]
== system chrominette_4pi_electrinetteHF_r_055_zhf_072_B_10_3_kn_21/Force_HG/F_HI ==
  In1 : Inport
  In2 : Inport  Port=2
  Add{19,22..23,41,49} (5 alike) : Sum
  Add2 : Sum  Inputs=+++
  Add24 : Sum  Inputs=+-
  Add26 : Sum  Inputs=-+
  Angle_Initial : Constant  Value=0
  C_100 : Constant  Value=-100
  Clock : Clock
  Constant1 : Constant  Value=10
  Constant{7..8,12,24} (4 alike) : Constant  Value=3
  Constant15 : Constant  Value=1.0E-3
  Constant2 : Constant  Value=1E-21
  Constant3 : Constant
  Constant4 : Constant  Value=2
  Constant5 : Constant  Value=2
  Math Function{1..3,16} (4 alike) : Math  Operator=square
  Math Function41 : Math  Operator=pow
  Math Function45 : Math  Operator=pow
  Math Function5 : Math  Operator=pow
  Nhix/Dhix2_3 : Scope
  Omega_w : Constant  Value=0.000005395168
  Product{4..5,7..8,11,19,30,71} (8 alike) : Product
  Product13 : Product  Inputs=**/
  Product14 : Product  Inputs=*/
  Product15 : Product  Inputs=*/
  Product16 : Product  Inputs=**
  Product18 : Product  Inputs=/*
  Product2 : Product  Inputs=/**
  Product23 : Product  Inputs=**
  Product3 : Product  Inputs=*/
  Product41 : Product  Inputs=**/
  Product6 : Product  Inputs=3
  Product68 : Product  Inputs=/**
  Sqrt : Sqrt
  Sqrt5 : Sqrt
  Sqrt6 : Sqrt
  Subtract : Sum
  Subtract1 : Sum  Inputs=+++
  Subtract2 : Sum  Inputs=+--
  Subtract6 : Sum
  Trigonometric Function1 : Trigonometry
  Trigonometric Function2 : Trigonometry  Operator=cos
  Trigonometric Function3 : Trigonometry
  Trigonometric Function4 : Trigonometry  Operator=cos
  Z0_1 : Constant  Value=0.321035617
  ex : Constant  Value=1.602176565
  k16x_2 : Constant  Value=0.505169378
  mh0x : Constant  Value=9.62404
  rx : Constant  Value=0.55605
  Out1 : Outport
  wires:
  Sqrt5/1 -> Product4/1  "sqrt(3)"
  Product3/1 -> Product4/2, Product7/2  "1/2"
  Constant15/1 -> Math Function45/1
  Sqrt6/1 -> Product30/1, Product14/1  "sqrt(3)"
  Product41/1 -> Product30/2, Subtract1/3  "r*cos(3wt)/2"
  Subtract/1 -> Product8/2
  Subtract2/1 -> Math Function16/1  "Z_hi"
  Trigonometric Function3/1 -> Product11/1  "sin(wt)"
  Constant7/1 -> Math Function5/2
  Product8/1 -> Product15/1
  Constant24/1 -> Math Function45/2
  Constant4/1 -> Product3/2
  Product13/1 -> Subtract1/2  "r*cos(wt)/2"
  Product2/1 -> Product71/2
  Product6/1 -> Subtract/2, Subtract2/1  "r*cos(wt)*sqrt(3)/2"
  Add41/1 -> Product71/1  "kn_Dhi"
  Product11/1 -> Add19/1  "r*sin(wt)"
  Subtract6/1 -> Product15/2
  Add24/1 -> Product18/2  "z - z0 + z3"
  Math Function41/1 -> Add41/1  "10_exp(-100Dhi/r)"
  Product18/1 -> Subtract2/2  "(z-z0+z3)/2"
  Product14/1 -> Product23/2  "sqrt(3)/2"
  Constant8/1 -> Sqrt6/1, Product19/2
  Product71/1 -> Product8/1
  Add2/1 -> Sqrt/1
  Angle_Initial/1 -> Add49/2
  Product4/1 -> Product6/1  "sqrt(3)/2"
  Z0_1/1 -> Add26/2  "Z0"
  Product23/1 -> Subtract1/1  "(z+z0-z3)*sqrt(3)/2"
  mh0x/1 -> Product2/1  "mx"
  Add22/1 -> Subtract/1  "z0 - z3 + z/2"
  Add49/1 -> Product19/1, Trigonometric Function4/1, Trigonometric Function3/1  "ai+wt"
  Add19/1 -> Math Function2/1  "r*sin(3wt) + r*sin(wt)"
  Subtract1/1 -> Math Function3/1  "X_hi"
  Omega_w/1 -> Product5/2
  Product19/1 -> Trigonometric Function2/1, Trigonometric Function1/1
  Add23/1 -> Product23/1  "z + z0 - z3"
  k16x_2/1 -> Product2/3
  Sqrt/1 -> Math Function5/1, Product68/3
  ex/1 -> Math Function1/1
  Math Function45/1 -> Subtract6/2
  Math Function1/1 -> Product2/2
  Product68/1 -> Math Function41/2
  Math Function16/1 -> Add2/3
  Constant3/1 -> Product3/1
  Trigonometric Function1/1 -> Product16/2  "sin(3wt)"
  Math Function5/1 -> Subtract6/1
  Constant12/1 -> Sqrt5/1
  Product16/1 -> Add19/2  "r*sin(3wt)"
  rx/1 -> Product6/3, Product68/1, Product13/2, Product41/2, Product16/1, Product11/2  "rx"
  Math Function3/1 -> Add2/2
  Product5/1 -> Add49/1  "angle_wt"
  Product15/1 -> Out1/1, Nhix/Dhix2_3/1  "nhix/dhix_3"
  Product30/1 -> Subtract2/3  "r*cos(3wt)*sqrt(3)/2"
  Math Function2/1 -> Add2/1
  Product7/1 -> Add22/2  "z/2"
  Trigonometric Function4/1 -> Product13/1, Product6/2  "cos(wt)"
  C_100/1 -> Product68/2
  Constant5/1 -> Product41/3, Product14/2, Product18/1, Product13/3  "2"
  Clock/1 -> Product5/1
  Trigonometric Function2/1 -> Product41/1  "cos(3wt)"
  In1/1 -> Product7/1, Add24/1, Add23/1
  Add26/1 -> Add22/1, Add23/2, Add24/2  "z0 - z3"
  In2/1 -> Add26/1
  Constant1/1 -> Math Function41/1
  Constant2/1 -> Add41/2

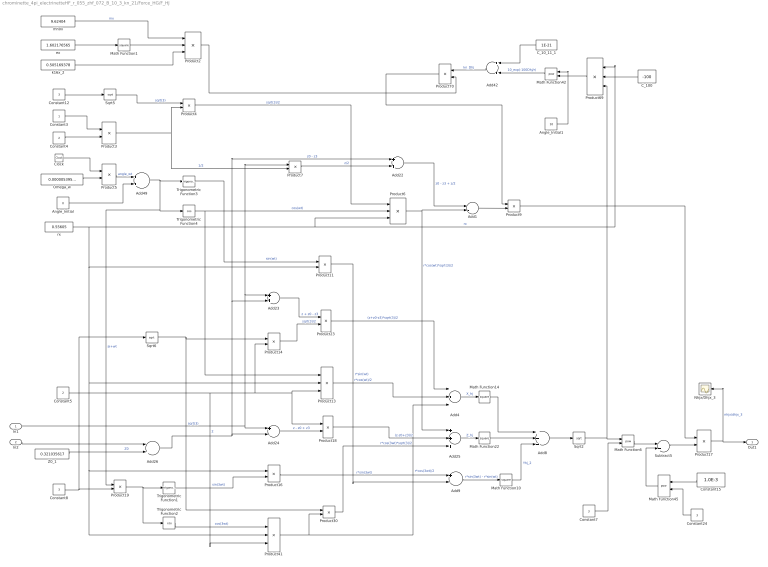
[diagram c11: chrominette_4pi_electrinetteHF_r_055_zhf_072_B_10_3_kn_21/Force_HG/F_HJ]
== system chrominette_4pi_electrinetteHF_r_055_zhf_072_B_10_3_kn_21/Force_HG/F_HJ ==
  In1 : Inport
  In2 : Inport  Port=2
  Add1 : Sum  Inputs=+-
  Add{22..23,42,49} (4 alike) : Sum
  Add24 : Sum  Inputs=+-
  Add25 : Sum  Inputs=+++
  Add26 : Sum  Inputs=-+
  Add4 : Sum  Inputs=-+-
  Add8 : Sum  Inputs=+++
  Add9 : Sum  Inputs=+-
  Angle_Initial : Constant  Value=0
  Angle_Initial1 : Constant  Value=10
  C_100 : Constant  Value=-100
  C_10_11_1 : Constant  Value=1E-21
  Clock : Clock
  Constant{7..8,12,24} (4 alike) : Constant  Value=3
  Constant15 : Constant  Value=1.0E-3
  Constant3 : Constant
  Constant4 : Constant  Value=2
  Constant5 : Constant  Value=2
  Math Function{1,10,14,22} (4 alike) : Math  Operator=square
  Math Function42 : Math  Operator=pow
  Math Function45 : Math  Operator=pow
  Math Function6 : Math  Operator=pow
  Nhjx/Dhjx_3 : Scope
  Omega_w : Constant  Value=0.000005395168
  Product{4..5,7,9,11,19,30,70} (8 alike) : Product
  Product13 : Product  Inputs=**/
  Product14 : Product  Inputs=*/
  Product16 : Product  Inputs=**
  Product17 : Product  Inputs=*/
  Product18 : Product  Inputs=/*
  Product2 : Product  Inputs=/**
  Product23 : Product  Inputs=**
  Product3 : Product  Inputs=*/
  Product41 : Product  Inputs=**/
  Product6 : Product  Inputs=3
  Product69 : Product  Inputs=/**
  Sqrt2 : Sqrt
  Sqrt5 : Sqrt
  Sqrt6 : Sqrt
  Subtract5 : Sum
  Trigonometric Function1 : Trigonometry
  Trigonometric Function2 : Trigonometry  Operator=cos
  Trigonometric Function3 : Trigonometry
  Trigonometric Function4 : Trigonometry  Operator=cos
  Z0_1 : Constant  Value=0.321035617
  ex : Constant  Value=1.602176565
  k16x_2 : Constant  Value=0.505169378
  mh0x : Constant  Value=9.62404
  rx : Constant  Value=0.55605
  Out1 : Outport
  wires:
  Product70/1 -> Product9/1
  Sqrt2/1 -> Product69/3, Math Function6/1
  Sqrt5/1 -> Product4/1  "sqrt(3)"
  Product3/1 -> Product4/2, Product7/2  "1/2"
  Constant15/1 -> Math Function45/1
  Sqrt6/1 -> Product14/1, Product30/1  "sqrt(3)"
  Product41/1 -> Product30/2, Add4/3  "r*cos(3wt)/2"
  Trigonometric Function3/1 -> Product11/1  "sin(wt)"
  Constant7/1 -> Math Function6/2
  Constant24/1 -> Math Function45/2
  Constant4/1 -> Product3/2
  Product13/1 -> Add4/2  "r*cos(wt)/2"
  Product2/1 -> Product70/2
  Product6/1 -> Add25/1, Add1/2  "r*cos(wt)*sqrt(3)/2"
  Product11/1 -> Add9/2  "r*sin(wt)"
  Add24/1 -> Product18/2  "z - z0 + z3"
  Product18/1 -> Add25/2  "(z-z0+z3)/2"
  Product14/1 -> Product23/2  "sqrt(3)/2"
  Math Function14/1 -> Add8/1
  Constant8/1 -> Sqrt6/1, Product19/2
  Angle_Initial/1 -> Add49/2
  Add4/1 -> Math Function14/1  "X_hj"
  Product4/1 -> Product6/1  "sqrt(3)/2"
  Product23/1 -> Add4/1  "(z+z0-z3)*sqrt(3)/2"
  mh0x/1 -> Product2/1  "mx"
  Add22/1 -> Add1/1  "z0 - z3 + z/2"
  Add49/1 -> Trigonometric Function3/1, Trigonometric Function4/1, Product19/1  "ai+wt"
  Product69/1 -> Math Function42/2
  Subtract5/1 -> Product17/2
  Omega_w/1 -> Product5/2
  Math Function22/1 -> Add8/2
  Product19/1 -> Trigonometric Function2/1, Trigonometric Function1/1
  Add23/1 -> Product23/1  "z + z0 - z3"
  Add42/1 -> Product70/1  "kn_Dhj"
  k16x_2/1 -> Product2/3
  Add25/1 -> Math Function22/1  "Z_hj"
  Math Function42/1 -> Add42/2  "10_exp(-100Dhj/r)"
  ex/1 -> Math Function1/1
  Math Function45/1 -> Subtract5/2
  Math Function6/1 -> Subtract5/1
  Math Function1/1 -> Product2/2
  Product17/1 -> Out1/1, Nhjx/Dhjx_3/1  "nhjx/dhjx_3"
  Add8/1 -> Sqrt2/1
  Constant3/1 -> Product3/1
  Trigonometric Function1/1 -> Product16/2  "sin(3wt)"
  Constant12/1 -> Sqrt5/1
  Product16/1 -> Add9/1  "r*sin(3wt)"
  Add1/1 -> Product9/2
  rx/1 -> Product13/2, Product41/2, Product16/1, Product11/2, Product6/3, Product69/1  "rx"
  Add9/1 -> Math Function10/1  "r*sin(3wt) - r*sin(wt)"
  Product5/1 -> Add49/1  "angle_wt"
  Product30/1 -> Add25/3  "r*cos(3wt)*sqrt(3)/2"
  Product7/1 -> Add22/2  "z/2"
  Trigonometric Function4/1 -> Product13/1, Product6/2  "cos(wt)"
  C_100/1 -> Product69/2
  Product9/1 -> Product17/1
  Constant5/1 -> Product41/3, Product14/2, Product13/3, Product18/1  "2"
  Math Function10/1 -> Add8/3  "Yhj_2"
  Clock/1 -> Product5/1
  Trigonometric Function2/1 -> Product41/1  "cos(3wt)"
  C_10_11_1/1 -> Add42/1
  In1/1 -> Product7/1, Add23/1, Add24/1
  Add26/1 -> Add22/1, Add23/2, Add24/2  "z0 - z3"
  Z0_1/1 -> Add26/2  "Z0"
  In2/1 -> Add26/1
  Angle_Initial1/1 -> Math Function42/1
